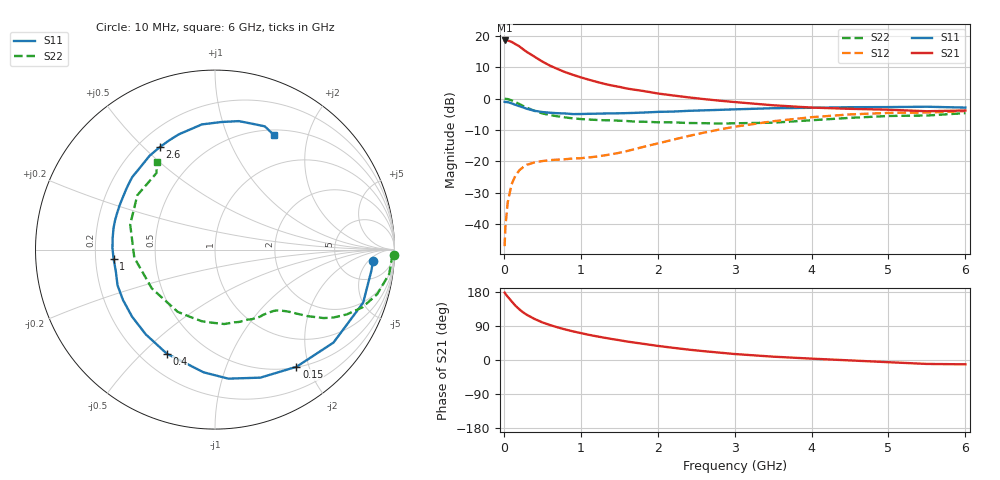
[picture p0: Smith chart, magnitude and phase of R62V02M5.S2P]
! SIEMENS Small Signal Semiconductors
! BFR193
! Si NPN RF Bipolar Junction Transistor in SOT23
! VCE = 2 V  IC = 2.5 mA
! Common Emitter S-Parameters:  May  1996
# GHz  S  MA  R  50
!  f  S11  S21  S12  S22
! GHz  MAG  ANG  MAG  ANG  MAG  ANG  MAG  ANG
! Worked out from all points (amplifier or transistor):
!   36 points, 10 MHz to 6 GHz, reference 50 ohm
!   highest |S21| = 18.5 dB at 10 MHz (marker M1)
!   |S21| within 3 dB of that: start of sweep to 261.7 MHz
!   unconditionally stable (mu >= 1): 1.076 GHz to 2.033 GHz
!   at 250 MHz: K = 0.27, MSG = 18.7 dB, |S12| = -21.8 dB
!   at 1.4 GHz: K = 1.10, MAG = 9.0 dB, |S12| = -17.7 dB
!   at 6 GHz: K = 0.99, MSG = 0.1 dB, |S12| = -4.0 dB
!   S11 on the Smith chart (normalised r, x): 10 MHz: 12, -7; 150 MHz: 0.51, -1.80; 400 MHz: 0.30, -0.60; 1 GHz: 0.28, -0.04; 2.6 GHz: 0.28, +0.56; 6 GHz: 0.57, +1.49
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0.01  0.8835 -4.0  8.375 177.8  0.0045 90.4  0.9974 -1.6
0.02  0.8787 -7.9  8.289 174.8  0.0091 85.9  0.986 -3.1
0.05  0.8769 -19.7  8.37 167.1  0.0223 79.7  0.9798 -8.0
0.1  0.8392 -38.1  7.971 155.1  0.0431 70.1  0.9368 -15.4
0.15  0.7953 -55.2  7.33 143.4  0.0595 61.9  0.882 -21.4
0.2  0.7568 -70.5  6.778 134.0  0.072 55.2  0.8195 -26.1
0.25  0.7228 -84.1  6.071 125.8  0.0811 49.4  0.7614 -29.8
0.3  0.6867 -95.3  5.486 119.1  0.0886 45.6  0.7158 -32.2
0.4  0.6388 -114.9  4.614 108.3  0.0966 40.0  0.6357 -35.7
0.5  0.6098 -129.2  3.872 99.3  0.1014 37.1  0.5802 -38.0
0.6  0.5942 -141.1  3.331 92.3  0.105 35.7  0.5461 -39.6
0.8  0.5783 -159.9  2.619 80.5  0.1085 35.9  0.5006 -42.8
1  0.5674 -174.9  2.171 71.0  0.1125 40.2  0.472 -46.5
1.1  0.5714 179.2  1.999 66.7  0.1157 42.4  0.4634 -49.0
1.3  0.5779 168.0  1.721 59.1  0.1244 47.5  0.4517 -53.6
1.6  0.5864 154.5  1.44 48.8  0.146 54.7  0.439 -62.0
2.2  0.6203 131.7  1.118 32.2  0.2216 60.2  0.4178 -82.9
2.6  0.6488 118.3  0.98 23.3  0.2865 57.9  0.4058 -100.5
3.5  0.7013 96.0  0.781 8.8  0.4351 43.2  0.4131 -148.4
4.5  0.728 79.5  0.686 -1.1  0.5586 23.4  0.4927 163.5
5.5  0.7406 68.0  0.628 -10.4  0.5987 5.0  0.5368 127.4
6  0.7176 62.7  0.645 -11.4  0.6326 -0.2  0.5862 123.5
